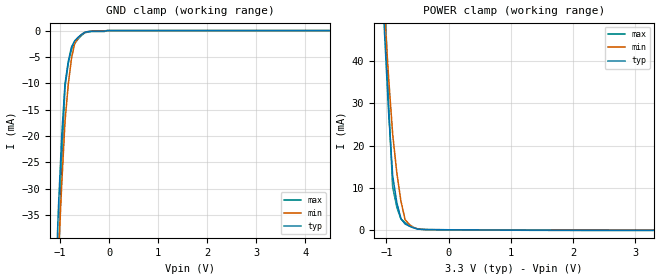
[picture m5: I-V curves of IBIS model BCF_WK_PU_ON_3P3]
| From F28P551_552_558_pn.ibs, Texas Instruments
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|BCF_RECEIVER_MODE_3P3; RECEIVER_MODE
|   Model Cell BCF_WK_PU_ON_3P3
|BCF_WK_PU_ON_3P3
[Model]   BCF_WK_PU_ON_3P3
Model_type   Input
Polarity   Non-Inverting
Vinl =  0.8
Vinh =  2
C_comp   1.28683p   1.00698p   1.46241p
[Model Spec]
Vinl   0.8   0.8   0.8
Vinh   2   2   2
[Temperature Range]   25   155   -40
[Voltage Range]   3.3   2.97   3.63
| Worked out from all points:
|   GND clamp passes 1 mA (typ) near -0.60 V on its own axis
|   POWER clamp passes 1 mA (typ) near -0.65 V on its own axis
| Nom Voltages:
|   BIASFET=3.3, VDD=1.2, VDDS=3.3, VSS=0
| Min Voltages:
|   BIASFET=2.97, VDD=1.08, VDDS=2.97, VSS=0
| Max Voltages:
|   BIASFET=3.63, VDD=1.32, VDDS=3.63, VSS=0
[POWER_clamp]
|   voltage   I(typ)   I(min)   I(max)
-3.3V     1.107A     1.023A     1.677A
-1.033V   47.41mA    52.06mA    58.67mA
-966.7mV  28.12mA    36.41mA    30.37mA
-900mV    12.83mA    22.69mA    10.14mA
-833.3mV  6.449mA    13.53mA    5.357mA
-766.7mV  2.627mA    6.766mA    2.544mA
-700mV    1.364mA    2.396mA    1.696mA
-633.3mV  862.5uA    1.277mA    1.079mA
-566.7mV  464.1uA    552.7uA    579.5uA
-500mV    169.1uA    223.1uA    198.3uA
-300mV    27.37uA    17.71uA    38.68uA
3.3V      -108.6uA   -62.32uA   -173.9uA
[GND_clamp]
|   voltage   I(typ)   I(min)   I(max)
-3.3V     -944.5mA   -826.8mA   -1.736A
-1.1V     -50.7mA    -57.86mA   -68.9mA
-1.033V   -33.49mA   -42.71mA   -43.83mA
-966.7mV  -19.96mA   -29.18mA   -24.42mA
-900mV    -10.12mA   -17.28mA   -10.68mA
-833.3mV  -5.823mA   -10.19mA   -6.218mA
-766.7mV  -3.088mA   -5.205mA   -3.458mA
-700mV    -1.914mA   -2.339mA   -2.395mA
-566.7mV  -751.8uA   -773.3uA   -957.3uA
-500mV    -334.3uA   -369.3uA   -429.8uA
-33.33mV  0A         0A         0A
6.6V      0A         0A         0A
